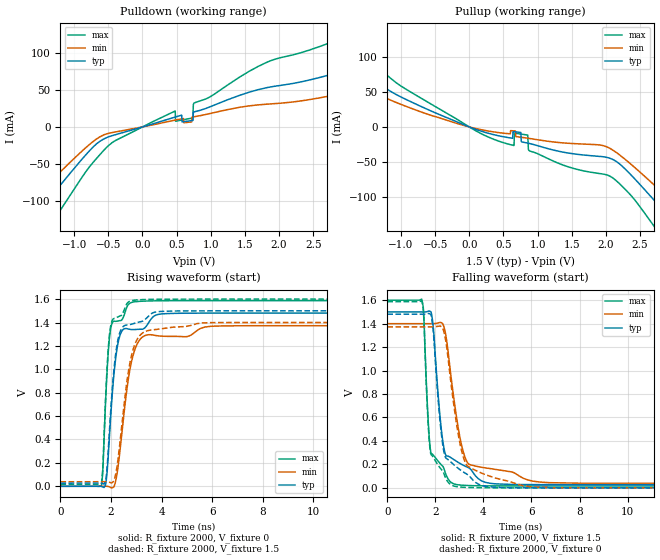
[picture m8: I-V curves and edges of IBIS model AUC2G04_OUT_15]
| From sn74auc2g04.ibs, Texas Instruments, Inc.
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[Model]   AUC2G04_OUT_15
Model_type  Output
Vref =   0
Rref =   2000
Cref =   15p
Vmeas =   0.75
| variable   typ   min   max
C_comp   6.42pF   1.69pF   19.05pF
| C_pullup   6.13pF   1.69pF   19.05pF
| C_pulldown   6.70pF   3.60pF   15.21pF
[Temperature Range]   40   100   -40
| Ambient temperature   25   85   -40
[Voltage range]   1.5   1.4   1.6
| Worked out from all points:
|   slope of the pulldown table from 0 to 0.225 V, typ, clamps not added: 36.6 ohm
|   slope of the pullup table from 0 to 0.225 V, typ, clamps not added: 29.5 ohm
|   rising waveform, R_fixture 2000, V_fixture 0: 20-80 % time 344ps typ, 508ps min, 228ps max; typ from 0 V to 1.48 V
|   falling waveform, R_fixture 2000, V_fixture 1.5: 20-80 % time 402ps typ, 608ps min, 236ps max; typ from 1.5 V to 0.027 V
|   rising waveform, R_fixture 2000, V_fixture 1.5: 20-80 % time 339ps typ, 501ps min, 225ps max; typ from 0.027 V to 1.5 V
|   falling waveform, R_fixture 2000, V_fixture 0: 20-80 % time 400ps typ, 614ps min, 234ps max; typ from 1.48 V to 0 V
[Pulldown]
| AUC2G04_OUT_15
|   Voltage   I(typ)   I(min)   I(max)
-3.6V     -343.2mA   -285.1mA   -423.9mA
-2.105V   -179.2mA   -144.2mA   -232.5mA
-1.795V   -144.8mA   -115.2mA   -192.1mA
-1.395V   -99.93mA   -78.06mA   -138.7mA
-395mV    -10.45mA   -6.753mA   -18.28mA
480mV     13.33mA    9.224mA    21.44mA
485mV     13.46mA    9.315mA    7.619mA
735mV     8.725mA    13.39mA    12.06mA
755mV     20.22mA    13.69mA    32.02mA
1.69V     50.07mA    29.62mA    81.22mA
3.34V     86.08mA    49.98mA    134.3mA
7.2V      80.6mA     45.5mA     141.2mA
[Pullup]
| AUC2G04_OUT_15
|   Voltage   I(typ)   I(min)   I(max)
-3.6V     253.3mA    194.5mA    303.7mA
-2.87V    186.5mA    147.2mA    232.6mA
-2.45V    149.4mA    116mA      191.5mA
-1.91V    104.2mA    79.12mA    139.3mA
100mV     -3.652mA   -2.395mA   -5.808mA
650mV     -6.722mA   -5.654mA   -26.6mA
855mV     -23.22mA   -16.17mA   -11.7mA
885mV     -23.88mA   -16.62mA   -34.51mA
2.105V    -46.98mA   -33.56mA   -73.62mA
2.76V     -111.3mA   -88.23mA   -150.2mA
3.37V     -179.4mA   -144.7mA   -232.4mA
7.2V      -606.3mA   -510.7mA   -734.4mA
[Ramp]
| AUC2G04_OUT_15
| variable   typ   min   max
dV/dt_r   0.89/3.46E-10   0.83/5.14E-10   0.95/2.30E-10
dV/dt_f   0.89/4.11E-10   0.82/6.10E-10   0.96/2.39E-10
R_load = 2000
[Rising Waveform]
| AUC2G04_OUT_15
R_fixture =   2000
C_fixture =   0
L_fixture =   0
V_fixture =   0
V_fixture_min = 0
V_fixture_max = 0
|   Time   V(typ)   V(min)   V(max)
0s        7.019nV    26.23nV    876.1pV
1.625ns   -1.674mV   511.3uV    7.385mV
1.805ns   37.42mV    481.4uV    813.4mV
1.98ns    570.2mV    -9.139mV   1.339V
2.135ns   997.5mV    7.353mV    1.412V
2.305ns   1.251V     212.2mV    1.414V
2.82ns    1.34V      1.074V     1.572V
3.33ns    1.353V     1.287V     1.583V
5.96ns    1.48V      1.368V     1.587V
22.2ns    1.481V     1.373V     1.587V
[Falling Waveform]
| AUC2G04_OUT_15
R_fixture =   2000
C_fixture =   0
L_fixture =   0
V_fixture =   1.5
V_fixture_min = 1.4
V_fixture_max = 1.6
|   Time   V(typ)   V(min)   V(max)
0s        1.5V       1.4V       1.6V
1.44ns    1.5V       1.4V       1.602V
1.515ns   1.5V       1.4V       1.475V
1.71ns    1.506V     1.4V       538.9mV
1.82ns    1.5V       1.399V     296.7mV
2.325ns   377.6mV    1.39V      179.3mV
2.78ns    239.7mV    745.7mV    33.51mV
3.375ns   172.3mV    205.2mV    19.94mV
6.06ns    27.74mV    57.26mV    16.5mV
22.2ns    27.2mV     38.79mV    16.41mV
[Rising Waveform]
| AUC2G04_OUT_15
R_fixture =   2000
C_fixture =   0
L_fixture =   0
V_fixture =   1.5
V_fixture_min = 1.4
V_fixture_max = 1.6
|   Time   V(typ)   V(min)   V(max)
0s        27.17mV    38.78mV    16.4mV
1.625ns   25.58mV    39.2mV     26.24mV
1.68ns    22.24mV    39.26mV    179mV
1.805ns   74.12mV    39.1mV     841.8mV
1.975ns   599.8mV    31.57mV    1.354V
2.28ns    1.258V     236mV      1.448V
2.755ns   1.383V     1.062V     1.583V
3.31ns    1.419V     1.319V     1.597V
5.6ns     1.5V       1.396V     1.6V
22.2ns    1.5V       1.4V       1.6V
[Falling Waveform]
| AUC2G04_OUT_15
R_fixture =   2000
C_fixture =   0
L_fixture =   0
V_fixture =   0
V_fixture_min = 0
V_fixture_max = 0
|   Time   V(typ)   V(min)   V(max)
0s        1.481V     1.373V     1.587V
1.435ns   1.48V      1.373V     1.591V
1.515ns   1.48V      1.373V     1.456V
1.715ns   1.486V     1.372V     495.6mV
1.82ns    1.475V     1.372V     284.5mV
2.305ns   369.4mV    1.361V     144mV
2.73ns    204.4mV    763.1mV    18.52mV
3.32ns    115.8mV    190.5mV    3.715mV
5.65ns    762.3uV    18.63mV    119.7uV
22.2ns    28.35uV    4.88uV     11.49uV
